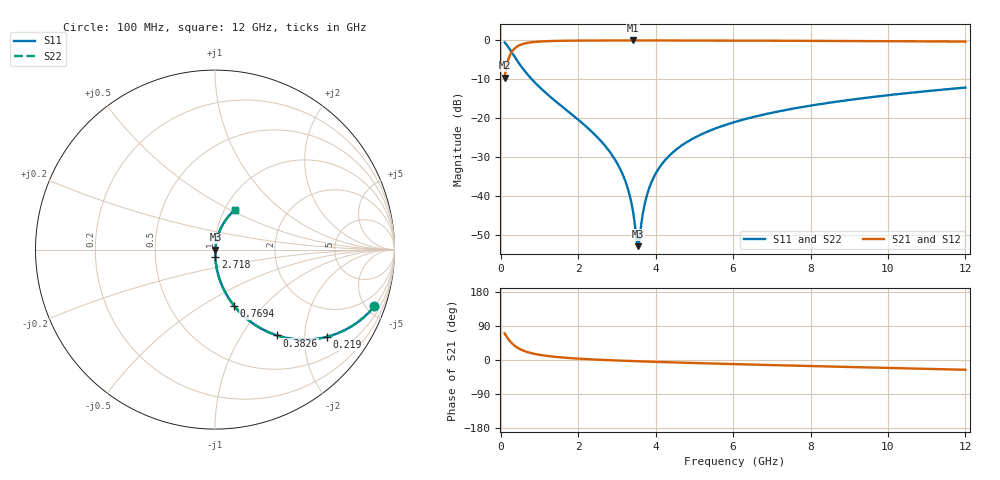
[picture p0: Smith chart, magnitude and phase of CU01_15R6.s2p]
! S-parameter model data by Modelithics Inc. support@modelithics.com 813-866-6335 Tampa FL USA
! S-Parameter data specifications:
! Substrate: 20-mil Rogers, substrate thickness, H=0.508mm, Dielectric constant, Er=3.75
! PCB Mounting Pad Footprint: Pad width, PadW=0.35mm , Pad length, PadL=0.30mm , Pad gap, PadG (edge-to-edge)=0.25mm , Reference planes=0.85mm apart
! Created Tue May  8 14:01:25 2018
# hz S ma R 50
! 2 Port Network Data from SP1.SP block
! freq  magS11  angS11  magS21  angS21  magS12  angS12  magS22  angS22
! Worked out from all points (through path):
!   801 points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, 100 MHz to 12 GHz, reference 50 ohm
!   highest |S21| = -0.02 dB at 3.417 GHz (marker M1); lowest = -9.6 dB at 100 MHz (marker M2)
!   group delay of S21, straight-line fit = 10.8 ps
!   lowest |S11| = -52.8 dB at 3.551 GHz (marker M3), VSWR 1.00, Z = 50.2 + j0.0117 ohm
!   |S11| at or under -10 dB: 805.7 MHz to end of sweep
!   |S22| runs from -52.8 to -0.5 dB; largest |S21 - S12| = 0
!   S11 on the Smith chart (normalised r, x): 100 MHz: 0.99, -5.64; 219 MHz: 0.99, -2.57; 382.6 MHz: 0.99, -1.46; 769.4 MHz: 0.99, -0.70; 2.718 GHz: 1.00, -0.09; 12 GHz: 1.12, +0.53
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1e8  0.9428 -19.5  0.3328 70.4  0.3328 70.4  0.9428 -19.5
2.19e8  0.7899 -38.0  0.6125 52.0  0.6125 52.0  0.7899 -38.0
3.82625e8  0.5904 -54.1  0.8062 35.8  0.8062 35.8  0.5904 -54.1
5.4625e8  0.4516 -63.5  0.8912 26.3  0.8912 26.3  0.4516 -63.5
7.69375e8  0.331 -71.2  0.9424 18.6  0.9424 18.6  0.331 -71.2
1.304875e9  0.1844 -80.1  0.9813 9.4  0.9813 9.4  0.1844 -80.1
2.09325e9  0.08787 -85.7  0.9943 3.0  0.9943 3.0  0.08787 -85.7
2.718e9  0.04303 -87.4  0.997 -0.1  0.997 -0.1  0.04303 -87.4
3.16425e9  0.01837 -85.2  0.9976 -2.0  0.9976 -2.0  0.01837 -85.2
3.313e9  0.01109 -81.0  0.9977 -2.5  0.9977 -2.5  0.01109 -81.0
3.417125e9  0.006317 -72.1  0.9977 -2.9  0.9977 -2.9  0.006317 -72.1
3.506375e9  0.002882 -41.2  0.9977 -3.2  0.9977 -3.2  0.002882 -41.2
3.551e9  0.002298 2.9  0.9977 -3.4  0.9977 -3.4  0.002298 2.9
3.58075e9  0.002789 31.2  0.9977 -3.5  0.9977 -3.5  0.002789 31.2
3.789e9  0.01091 73.4  0.9975 -4.2  0.9975 -4.2  0.01091 73.4
4.071625e9  0.02239 78.7  0.9973 -5.2  0.9973 -5.2  0.02239 78.7
4.384e9  0.0344 79.7  0.9969 -6.1  0.9969 -6.1  0.0344 79.7
4.8005e9  0.04944 79.6  0.9961 -7.4  0.9961 -7.4  0.04944 79.6
6.05e9  0.08998 77.3  0.993 -10.9  0.993 -10.9  0.08998 77.3
8.04325e9  0.1468 72.6  0.9858 -16.1  0.9858 -16.1  0.1468 72.6
1.002162e10  0.1986 68.0  0.9763 -21.0  0.9763 -21.0  0.1986 68.0
1.2e10  0.2482 63.3  0.9645 -25.8  0.9645 -25.8  0.2482 63.3
